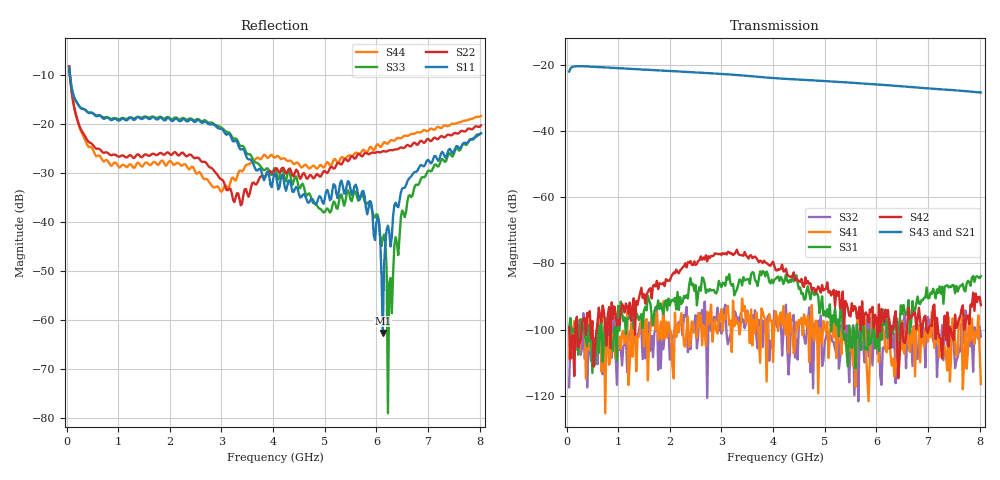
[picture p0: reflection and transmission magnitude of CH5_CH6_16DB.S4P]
!Agilent Technologies,E5071C,MY46316741,A.11.02
!Date: Mon Jun 01 10:41:27 2026
!Data & Calibration Information:
!1:CH5 INPUT 2:CH5 OUTPUT 3:CH6 INPUT 4:CH6 OUTPUT
!Freq	S11:SOLT4(ON)	S12:SOLT4(ON)	S13:SOLT4(ON)	S14:SOLT4(ON)
!	S21:SOLT4(ON)	S22:SOLT4(ON)	S23:SOLT4(ON)	S24:SOLT4(ON)
!	S31:SOLT4(ON)	S32:SOLT4(ON)	S33:SOLT4(ON)	S34:SOLT4(ON)
!	S41:SOLT4(ON)	S42:SOLT4(ON)	S43:SOLT4(ON)	S44:SOLT4(ON)
!PortZ  Port1:50+j0  Port2:50+j0  Port3:50+j0  Port4:50+j0
!Above PortZ is port z conversion or system Z0 setting when saving the data.
!When reading, reference impedance value at option line is always used.
# Hz S dB R 50
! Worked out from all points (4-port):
!   320 points, 50 MHz to 8.025 GHz, reference 50 ohm
!   strongest paths, dB at 50 MHz, 2.05 GHz, 4.05 GHz, 6.05 GHz, 8.025 GHz:
!     S43: -21.9, -21.7, -23.9, -25.8, -28.2
!     S21: -21.9, -21.9, -24.1, -26.1, -28.5
!     S42: -99.3, -83.4, -82.0, -92.4, -92.6
!     S31: -99.8, -90.9, -84.7, -106.6, -83.8
!     S41: -108.8, -111.0, -94.6, -109.9, -116.5
!     S32: -117.5, -102.5, -97.7, -100.0, -102.1
!   lowest |S11| = -62.7 dB at 6.125 GHz (marker M1), VSWR 1.00, Z = 50.1 - j0.0369 ohm
!   |S11| at or under -10 dB: 63.83 MHz to end of sweep
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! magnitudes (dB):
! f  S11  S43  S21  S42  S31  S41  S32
! 50 MHz  -8.6  -21.9  -21.9  -99.3  -99.8  -108.8  -117.5
! 5.75 GHz  -33.7  -25.5  -25.7  -98.5  -97.9  -103.6  -106.1
! 6.125 GHz  -62.7  -25.9  -26.2  -95.8  -93.9  -97.5  -105.5
! 6.225 GHz  -40.8  -26.0  -26.3  -94.1  -102.6  -104.5  -99.2
! 6.25 GHz  -42.1  -26.1  -26.3  -98.6  -97.7  -96.8  -105.8
! 6.5 GHz  -33.2  -26.4  -26.6  -98.1  -95.3  -97.3  -105.3
! 8.025 GHz  -22.0  -28.2  -28.5  -92.6  -83.8  -116.5  -102.1
